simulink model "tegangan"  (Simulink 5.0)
settings: Solver=ode45  StartTime=0.0  StopTime=3  RelTol=1e-3
libraries: simulink x2

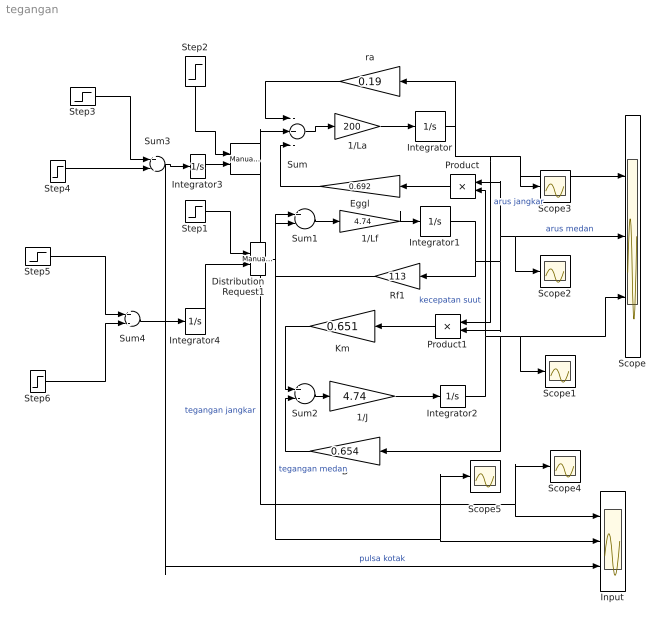
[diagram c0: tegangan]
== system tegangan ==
  " " : simulink/Signal Routing/Manual Switch  sw=0  action=0
  1/J : Gain  Gain=4.74
  1/La : Gain  Gain=200
  1/Lf : Gain  Gain=4.74
  B : Gain  Orientation=left  Gain=0.654
  Distribution Request1 : simulink/Signal Routing/Manual Switch  sw=1  action=0
  Eggl : Gain  Orientation=left  Gain=0.692
  Input : Scope  NumInputPorts=3
  Integrator{,1..4} (5 alike) : Integrator
  Km : Gain  Orientation=left  Gain=0.651
  Product : Product  Orientation=left
  Product1 : Product  Orientation=left
  Rf1 : Gain  Orientation=left  Gain=113
  Scope : Scope  NumInputPorts=3
  Scope{1..5} (5 alike) : Scope
  Step1 : Step  Time=0  After=300  SampleTime=0
  Step2 : Step  Orientation=down  Time=0  After=500  SampleTime=0
  Step3 : Step  Time=0  After=500  SampleTime=0
  Step4 : Step  After=500  SampleTime=0
  Step5 : Step  Time=0  After=300  SampleTime=0
  Step6 : Step  Time=0.998  After=300  SampleTime=0
  Sum : Sum  Inputs=-+-
  Sum{1..4} (4 alike) : Sum  Inputs=+-
  ra : Gain  Orientation=left  Gain=0.19
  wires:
  Sum/1 -> 1/La/1
  1/La/1 -> Integrator/1
  Integrator/1 -> ra/1, Product1/1, Scope/1, Scope3/1  "arus jangkar"
  Product/1 -> Eggl/1
  Sum1/1 -> 1/Lf/1
  1/Lf/1 -> Integrator1/1
  Integrator1/1 -> Product1/2, Product/1, Scope/2, Scope2/1, Rf1/1  "arus medan"
  1/J/1 -> Integrator2/1
  Product1/1 -> Km/1
  B/1 -> Sum2/2
  Km/1 -> Sum2/1
  Eggl/1 -> Sum/3
  Step1/1 -> Distribution Request1/1
  Integrator3/1 -> " "/2
  ra/1 -> Sum/1
  Step3/1 -> Sum3/1
  Step6/1 -> Sum4/2
  Sum2/1 -> 1/J/1
  Integrator2/1 -> B/1, Scope/3, Scope1/1, Product/2  "kecepatan suut"
  Rf1/1 -> Sum1/2
  Sum3/1 -> Integrator3/1, Input/3  "pulsa kotak"
  Sum4/1 -> Integrator4/1
  Step4/1 -> Sum3/2
  Step5/1 -> Sum4/1
  Step2/1 -> " "/1
  Distribution Request1/1 -> Sum1/1, Input/2, Scope5/1  "tegangan medan"
  Integrator4/1 -> Distribution Request1/2
  " "/1 -> Sum/2, Input/1, Scope4/1  "tegangan jangkar"
